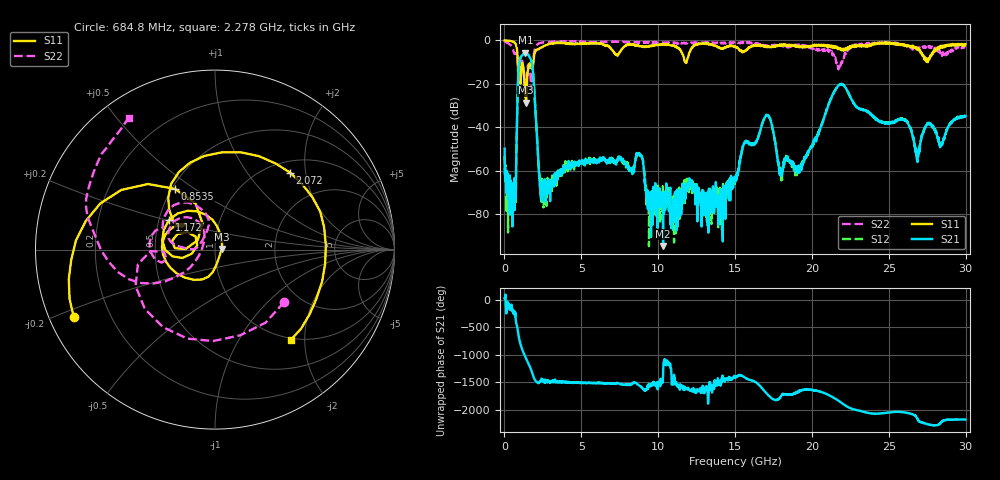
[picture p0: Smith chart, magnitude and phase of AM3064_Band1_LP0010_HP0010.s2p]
# Hz S DB R 50.0
!freq dBS11 angS11 dBS21 angS21 dBS12 angS12 dBS22 angS22
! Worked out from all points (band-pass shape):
!   1600 points, 10 MHz to 29.98 GHz, reference 50 ohm
!   highest |S21| = -5.66 dB at 1.36 GHz (marker M1); lowest = -94.6 dB at 10.32 GHz (marker M2)
!   |S21| within 3 dB of the highest: 1.016 GHz to 1.714 GHz (697.9 MHz wide, 51.1 % of centre)
!   lowest |S11| = -28.6 dB at 1.397 GHz (marker M3), VSWR 1.08, Z = 53.8 + j0.388 ohm
!   |S11| at or under -10 dB: 865.6 MHz to 1.877 GHz (1.011 GHz wide, 73.7 % of centre); 11.75 GHz to 11.84 GHz (92.77 MHz wide, 0.786 % of centre)
!   |S22| runs from -22.8 to -0.2 dB; largest |S21 - S12| = 0.0062
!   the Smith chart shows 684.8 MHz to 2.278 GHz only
!   S11 on the Smith chart (normalised r, x): 684.8 MHz: 0.07, -0.22; 853.5 MHz: 0.52, +0.42; 1.172 GHz: 0.57, +0.21; 2.072 GHz: 1.23, +1.64; 2.278 GHz: 0.96, -1.71
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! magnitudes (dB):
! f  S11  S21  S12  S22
! 10 MHz  0.0  -49.8  -53.1  -0.2
! 684.8 MHz  -1.2  -67.5  -64.7  -6.3
! 853.5 MHz  -7.9  -25.1  -25.0  -8.9
! 1.172 GHz  -10.3  -6.7  -6.6  -9.8
! 1.36 GHz  -25.4  -5.7  -5.7  -21.0
! 1.397 GHz  -28.6  -5.7  -5.7  -19.1
! 1.772 GHz  -12.8  -10.2  -10.1  -20.4
! 2.072 GHz  -4.4  -39.1  -39.3  -2.3
! 2.278 GHz  -3.6  -62.4  -62.4  -1.2
! 5.015 GHz  -1.4  -56.3  -55.9  -0.7
! 8.782 GHz  -2.7  -52.7  -53.0  -0.9
! 9.363 GHz  -2.8  -71.2  -72.0  -1.0
! 10 GHz  -2.0  -71.3  -75.5  -0.9
! 10.32 GHz  -1.9  -94.6  -70.5  -1.0
! 15 GHz  -3.0  -64.4  -63.8  -1.3
! 17.05 GHz  -2.9  -34.4  -34.4  -2.7
! 17.99 GHz  -2.4  -61.4  -62.9  -2.4
! 19.99 GHz  -2.7  -48.4  -49.0  -3.4
! 21.85 GHz  -3.5  -20.2  -20.0  -12.5
! 25 GHz  -1.0  -38.4  -37.9  -1.2
! 26.85 GHz  -4.2  -55.5  -54.3  -3.2
! 29.98 GHz  -1.8  -34.8  -35.2  -3.2
